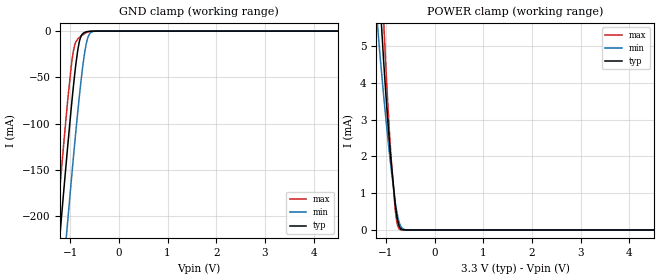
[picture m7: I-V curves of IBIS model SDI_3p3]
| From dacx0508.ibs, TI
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|   Model
[Model]   SDI_3p3
Model_type   Input
Vinl = 0.99
Vinh = 2.31
|   typ   min   max
C_comp   1.1367pF   1.0319pF   1.1793pF
| Where nom  PVT is Nominal Process, 3.3V, 27C
|   Fast PVT is Strong Process,  3.6V, -40C
|   Slow PVT is Weak Process,   3.0V, 125C
[Voltage Range]   3.3   3   3.6
|Junction Temperature
[Temperature Range]   27   125   -40
[Power Clamp Reference]   3.3   3   3.6
[GND Clamp Reference]   0   0   0
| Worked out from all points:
|   GND clamp passes 1 mA (typ) near -0.68 V on its own axis
|   POWER clamp passes 1 mA (typ) near -0.83 V on its own axis
[GND Clamp]
|   Voltage   I(typ)   I(min)   I(max)
-3.3V     -1.579A    -1.657A    -1.531A
-1.33V    -295.1mA   -377.4mA   -243.3mA
-1.201V   -214.9mA   -297.1mA   -163.2mA
-1.073V   -137.1mA   -218.4mA   -86.92mA
-983.4mV  -86.09mA   -165.4mA   -40.53mA
-933.9mV  -59.77mA   -136.7mA   -21.52mA
-884.4mV  -36.2mA    -109mA     -11.74mA
-815.1mV  -12.21mA   -72.23mA   -7.091mA
-696.3mV  -1.319mA   -21.27mA   -2.532mA
-607.2mV  -256.1uA   -3.549mA   -604.4uA
-468.6mV  -8.55uA    -84.23uA   -13.72uA
6.6V      0A         0A         0A
[POWER Clamp]
|   Voltage   I(typ)   I(min)   I(max)
-3.3V     65.24mA    51.4mA     78.94mA
-1.171V   7.367mA    5.513mA    9.303mA
-1.122V   6.192mA    4.72mA     7.805mA
-1.053V   4.657mA    3.7mA      5.779mA
-1.043V   4.452mA    3.561mA    5.499mA
-933.9mV  2.455mA    2.122mA    2.732mA
-904.2mV  1.979mA    1.759mA    2.109mA
-815.1mV  744uA      797.4uA    598.6uA
-765.6mV  280.2uA    399.3uA    138.7uA
-706.2mV  45.78uA    120.4uA    9.747uA
-498.3mV  24.78nA    350.1nA    0A
6.6V      0A         0A         0A
